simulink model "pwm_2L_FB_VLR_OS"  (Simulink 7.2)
settings: Solver=ode3  SolverMode=SingleTasking  StartTime=0.0  StopTime=0.1  FixedStep=10e-6  MaxStep=1e-4  RelTol=1e-3
PreLoadFcn:
  | INIT_PWM_2L

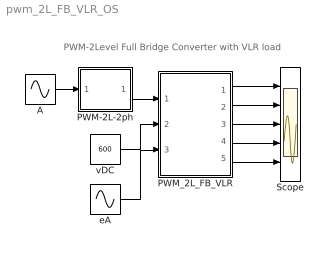
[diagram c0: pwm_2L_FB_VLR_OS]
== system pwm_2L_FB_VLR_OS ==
  note: PWM-2Level Full Bridge Converter with VLR load
  A : Sin  Amplitude=.8  Frequency=2*pi*50  Phase=[0 ]  SampleTime=0
  PWM-2L-2ph : Subsystem  mask(PWM-2L-2PH){FT=900, PHT=0, DT=1e-6}
      mask prompts: FT "Triangular Frequency"; PHT "Trian. Phase Angle (Degree)"; DT "Dead Time"
      mask help: Pulse Width Modulation for 2 Legs of 2-Level Converter
  PWM_2L_FB_VLR : Subsystem  mask(pwm_2L_FB_VLR_OS){RL=1, LL=1e-3}
      mask prompts: RL "Load R"; LL "Load L"
      mask help: Open Source 2-Level FB_PWM Converter with VLR load Input Vector u: u[0]= TD1.gate u[1]= TD2.gate u[2]= TD3.gate u[3]= TD4.gate u[4]= VDC u[5]= EL, Load Voltage Output Vector y: y[0]= Va.v, Output Voltage to middle point y[1]= Ia.I, Output AC Current y[2]= Vab.V, Output AC Voltage y[3]= T1.I y[4]= D1.I y[5]= T1.V y[6]= DC.I, Input DC Current Parameter Vector p: p[0]= RL p[1]= LL You can pause the simulation during running, change the Parameters you want and continue the Simulation
  Scope : Scope  NumInputPorts=5
  eA : Sin  Amplitude=100  Frequency=2*pi*50  Phase="[0  ]"  SampleTime=0
  vDC : Constant  Value=600  OutDataType=sfix(16)  OutScaling=2^0
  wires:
  A/1 -> PWM-2L-2ph/1(I1)
  PWM_2L_FB_VLR/1(vA) -> Scope/1
  vDC/1 -> PWM_2L_FB_VLR/2(vDC)
  PWM-2L-2ph/1(O1) -> PWM_2L_FB_VLR/1(Sw)
  eA/1 -> PWM_2L_FB_VLR/3(EA)
  PWM_2L_FB_VLR/2(iA1) -> Scope/2
  PWM_2L_FB_VLR/3(vAB) -> Scope/3
  PWM_2L_FB_VLR/4(iT1,iD1,vT1) -> Scope/4
  PWM_2L_FB_VLR/5(iDC) -> Scope/5

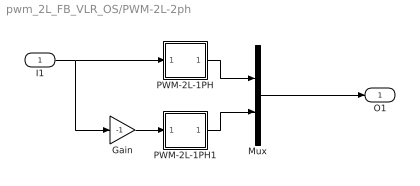
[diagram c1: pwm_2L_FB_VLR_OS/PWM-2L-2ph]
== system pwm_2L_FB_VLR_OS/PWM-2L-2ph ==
  I1 : Inport  OutDataType=sfix(16)  OutScaling=2^0
  Gain : Gain  Gain=-1  ParameterDataType=sfix(16)  ParameterScaling=2^0  OutDataType=sfix(16)  OutScaling=2^0
  Mux : Mux  Inputs=2
  PWM-2L-1PH : Subsystem  mask(PWM-2L-1PH){FT=FT, PHT=PHT, DT=DT}
      mask prompts: FT "Triangular Frequency"; PHT "Trian. Phase Angle (Degree)"; DT "Dead Time"
      mask help: Pulse Width Modulation for 1 Phase Converter
  PWM-2L-1PH1 : Subsystem  mask(PWM-2L-1PH){FT=FT, PHT=PHT, DT=DT}
      mask prompts: FT "Triangular Frequency"; PHT "Trian. Phase Angle (Degree)"; DT "Dead Time"
      mask help: Pulse Width Modulation for 1 Phase Converter
  O1 : Outport
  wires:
  Gain/1 -> PWM-2L-1PH1/1(In1)
  I1/1 -> Gain/1, PWM-2L-1PH/1(In1)
  PWM-2L-1PH/1(Out1) -> Mux/1
  PWM-2L-1PH1/1(Out1) -> Mux/2
  Mux/1 -> O1/1

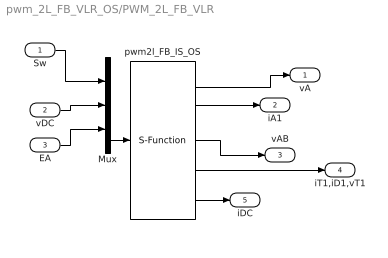
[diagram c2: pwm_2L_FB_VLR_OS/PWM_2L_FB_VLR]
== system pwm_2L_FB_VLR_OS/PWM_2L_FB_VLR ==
  Sw : Inport  OutDataType=sfix(16)  OutScaling=2^0
  vDC : Inport  Port=2  OutDataType=sfix(16)  OutScaling=2^0
  EA : Inport  Port=3  OutDataType=sfix(16)  OutScaling=2^0
  Mux : Mux  Inputs="[4  1  1]"
  pwm2l_FB_IS_OS : S-Function  FunctionName=s_pwm_2L_FB_VLR_OS  Parameters="[RL  LL]"  EnableBusSupport=off
  vA : Outport  OutDataType=sfix(16)  OutScaling=2^0
  iA1 : Outport  Port=2  OutDataType=sfix(16)  OutScaling=2^0
  vAB : Outport  Port=3  OutDataType=sfix(16)  OutScaling=2^0
  iT1,iD1,vT1 : Outport  Port=4  OutDataType=sfix(16)  OutScaling=2^0
  iDC : Outport  Port=5  OutDataType=sfix(16)  OutScaling=2^0
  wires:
  pwm2l_FB_IS_OS/4 -> iT1,iD1,vT1/1
  pwm2l_FB_IS_OS/3 -> vAB/1
  pwm2l_FB_IS_OS/2 -> iA1/1
  pwm2l_FB_IS_OS/1 -> vA/1
  EA/1 -> Mux/3
  Mux/1 -> pwm2l_FB_IS_OS/1
  vDC/1 -> Mux/2
  Sw/1 -> Mux/1
  pwm2l_FB_IS_OS/5 -> iDC/1

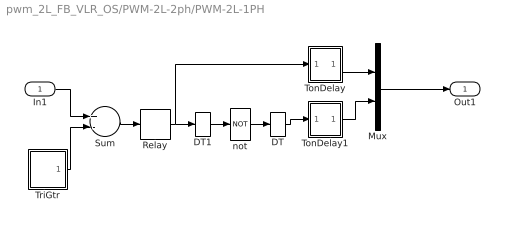
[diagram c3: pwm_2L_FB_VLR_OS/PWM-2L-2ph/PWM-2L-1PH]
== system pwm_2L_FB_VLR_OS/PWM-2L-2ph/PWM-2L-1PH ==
  In1 : Inport  OutDataType=sfix(16)  OutScaling=2^0
  DT : DataTypeConversion
  DT1 : DataTypeConversion
  Mux : Mux  Inputs=2
  Relay : Relay  OutDataType=sfix(16)  OutScaling=2^0
  Sum : Sum  Inputs=+-  OutDataType=sfix(16)  OutScaling=2^0
  TonDelay : Subsystem  mask(TonDelay){DT=DT}
      mask prompts: DT "Dead Time"
      mask help: Turn on dead time to protect against short circuit of the converter leg
  TonDelay1 : Subsystem  mask(TonDelay){DT=DT}
      mask prompts: DT "Dead Time"
      mask help: Turn on dead time to protect against short circuit of the converter leg
  TriGtr : Subsystem  mask(TriGtr){T=1/FT, Td=PHT/FT/360}
      mask prompts: T "Period Time"; Td "Time Delay"
      mask help: Triangular Wave Generator with variable time delay
  not : Logic  Operator=NOT  Inputs=1
  Out1 : Outport  InitialOutput=0
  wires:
  DT1/1 -> not/1
  DT/1 -> TonDelay1/1(s1)
  In1/1 -> Sum/1
  TriGtr/1(O) -> Sum/2
  Sum/1 -> Relay/1
  not/1 -> DT/1
  TonDelay1/1(s1d) -> Mux/2
  Relay/1 -> DT1/1, TonDelay/1(s1)
  TonDelay/1(s1d) -> Mux/1
  Mux/1 -> Out1/1

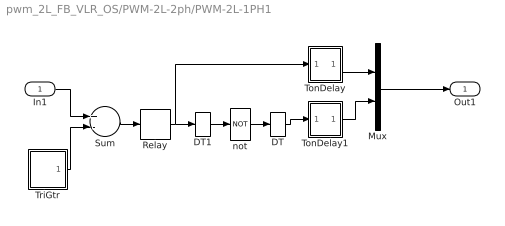
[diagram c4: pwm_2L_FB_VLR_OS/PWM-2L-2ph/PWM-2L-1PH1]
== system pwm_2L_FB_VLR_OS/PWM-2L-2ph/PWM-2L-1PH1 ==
  In1 : Inport  OutDataType=sfix(16)  OutScaling=2^0
  DT : DataTypeConversion
  DT1 : DataTypeConversion
  Mux : Mux  Inputs=2
  Relay : Relay  OutDataType=sfix(16)  OutScaling=2^0
  Sum : Sum  Inputs=+-  OutDataType=sfix(16)  OutScaling=2^0
  TonDelay : Subsystem  mask(TonDelay){DT=DT}
      mask prompts: DT "Dead Time"
      mask help: Turn on dead time to protect against short circuit of the converter leg
  TonDelay1 : Subsystem  mask(TonDelay){DT=DT}
      mask prompts: DT "Dead Time"
      mask help: Turn on dead time to protect against short circuit of the converter leg
  TriGtr : Subsystem  mask(TriGtr){T=1/FT, Td=PHT/FT/360}
      mask prompts: T "Period Time"; Td "Time Delay"
      mask help: Triangular Wave Generator with variable time delay
  not : Logic  Operator=NOT  Inputs=1
  Out1 : Outport  InitialOutput=0
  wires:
  Mux/1 -> Out1/1
  TonDelay/1(s1d) -> Mux/1
  Relay/1 -> TonDelay/1(s1), DT1/1
  TonDelay1/1(s1d) -> Mux/2
  not/1 -> DT/1
  Sum/1 -> Relay/1
  TriGtr/1(O) -> Sum/2
  In1/1 -> Sum/1
  DT/1 -> TonDelay1/1(s1)
  DT1/1 -> not/1

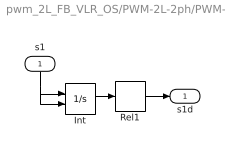
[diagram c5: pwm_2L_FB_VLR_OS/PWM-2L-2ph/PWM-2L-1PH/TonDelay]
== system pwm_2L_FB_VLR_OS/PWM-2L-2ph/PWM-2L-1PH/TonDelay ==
  s1 : Inport  Orientation=down  OutDataType=sfix(16)  OutScaling=2^0
  Int : Integrator  ExternalReset=falling
  Rel1 : Relay  OnSwitchValue=DT  OutDataType=sfix(16)  OutScaling=2^0
  s1d : Outport  InitialOutput=0
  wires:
  Int/1 -> Rel1/1
  s1/1 -> Int/2, Int/1
  Rel1/1 -> s1d/1

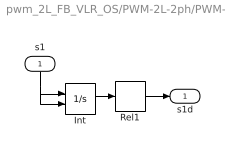
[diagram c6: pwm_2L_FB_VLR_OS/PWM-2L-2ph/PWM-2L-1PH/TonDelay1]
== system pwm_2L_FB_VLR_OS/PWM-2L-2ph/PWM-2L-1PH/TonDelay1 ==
  s1 : Inport  Orientation=down  OutDataType=sfix(16)  OutScaling=2^0
  Int : Integrator  ExternalReset=falling
  Rel1 : Relay  OnSwitchValue=DT  OutDataType=sfix(16)  OutScaling=2^0
  s1d : Outport  InitialOutput=0
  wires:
  Int/1 -> Rel1/1
  s1/1 -> Int/2, Int/1
  Rel1/1 -> s1d/1

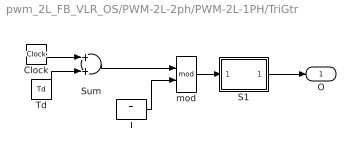
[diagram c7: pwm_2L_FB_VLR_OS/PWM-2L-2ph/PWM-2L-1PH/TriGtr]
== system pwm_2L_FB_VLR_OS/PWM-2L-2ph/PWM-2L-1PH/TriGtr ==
  Clock : Clock
  S1 : Subsystem
  Sum : Sum  OutDataType=sfix(16)  OutScaling=2^0
  T : Constant  Value=T  OutDataType=sfix(16)  OutScaling=2^0
  Td : Constant  Value=Td  OutDataType=sfix(16)  OutScaling=2^0
  mod : Math  Operator=mod
  O : Outport  InitialOutput=0
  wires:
  mod/1 -> S1/1(I1)
  S1/1(O1) -> O/1
  Clock/1 -> Sum/1
  T/1 -> mod/2
  Sum/1 -> mod/1
  Td/1 -> Sum/2

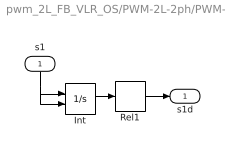
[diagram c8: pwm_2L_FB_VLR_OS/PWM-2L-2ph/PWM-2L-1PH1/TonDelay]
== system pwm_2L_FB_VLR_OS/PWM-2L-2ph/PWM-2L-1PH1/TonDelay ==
  s1 : Inport  Orientation=down  OutDataType=sfix(16)  OutScaling=2^0
  Int : Integrator  ExternalReset=falling
  Rel1 : Relay  OnSwitchValue=DT  OutDataType=sfix(16)  OutScaling=2^0
  s1d : Outport  InitialOutput=0
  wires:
  Rel1/1 -> s1d/1
  s1/1 -> Int/1, Int/2
  Int/1 -> Rel1/1

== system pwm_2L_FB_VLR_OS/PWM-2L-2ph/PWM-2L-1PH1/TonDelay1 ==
  s1 : Inport  Orientation=down  OutDataType=sfix(16)  OutScaling=2^0
  Int : Integrator  ExternalReset=falling
  Rel1 : Relay  OnSwitchValue=DT  OutDataType=sfix(16)  OutScaling=2^0
  s1d : Outport  InitialOutput=0
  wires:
  Rel1/1 -> s1d/1
  s1/1 -> Int/1, Int/2
  Int/1 -> Rel1/1

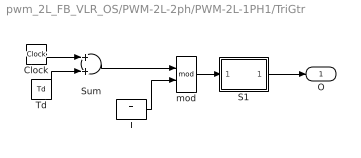
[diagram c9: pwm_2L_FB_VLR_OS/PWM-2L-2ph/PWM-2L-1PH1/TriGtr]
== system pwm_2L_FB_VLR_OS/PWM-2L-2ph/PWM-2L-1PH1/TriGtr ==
  Clock : Clock
  S1 : Subsystem
  Sum : Sum  OutDataType=sfix(16)  OutScaling=2^0
  T : Constant  Value=T  OutDataType=sfix(16)  OutScaling=2^0
  Td : Constant  Value=Td  OutDataType=sfix(16)  OutScaling=2^0
  mod : Math  Operator=mod
  O : Outport  InitialOutput=0
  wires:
  Td/1 -> Sum/2
  Sum/1 -> mod/1
  T/1 -> mod/2
  Clock/1 -> Sum/1
  S1/1(O1) -> O/1
  mod/1 -> S1/1(I1)

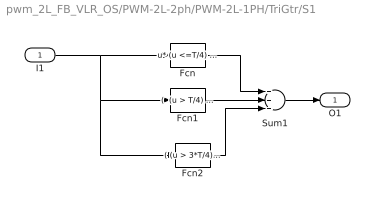
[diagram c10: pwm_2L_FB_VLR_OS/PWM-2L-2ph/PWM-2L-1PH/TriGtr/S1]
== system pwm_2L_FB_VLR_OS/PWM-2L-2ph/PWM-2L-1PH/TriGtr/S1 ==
  I1 : Inport  OutDataType=sfix(16)  OutScaling=2^0
  Fcn : Fcn  Expr=u* (u <=T/4) * 4/T
  Fcn1 : Fcn  Expr="(  (u > T/4) && ( u <=3*T/4) )* ( 1 - (u-T/4) *4/T )"
  Fcn2 : Fcn  Expr=( (u > 3*T/4)&& (u<=T)) * ( ((u -3*T/4)* 4/T )-1 )
  Sum1 : Sum  Inputs=+++  OutDataType=sfix(16)  OutScaling=2^0
  O1 : Outport
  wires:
  Fcn2/1 -> Sum1/3
  Fcn1/1 -> Sum1/2
  Fcn/1 -> Sum1/1
  Sum1/1 -> O1/1
  I1/1 -> Fcn/1, Fcn2/1, Fcn1/1

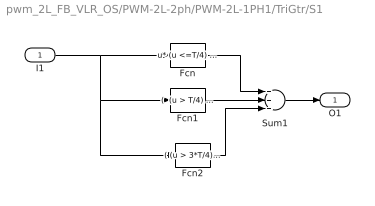
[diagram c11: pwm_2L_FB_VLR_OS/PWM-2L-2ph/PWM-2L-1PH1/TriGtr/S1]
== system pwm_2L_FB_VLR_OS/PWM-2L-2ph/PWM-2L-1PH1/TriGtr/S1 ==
  I1 : Inport  OutDataType=sfix(16)  OutScaling=2^0
  Fcn : Fcn  Expr=u* (u <=T/4) * 4/T
  Fcn1 : Fcn  Expr="(  (u > T/4) && ( u <=3*T/4) )* ( 1 - (u-T/4) *4/T )"
  Fcn2 : Fcn  Expr=( (u > 3*T/4)&& (u<=T)) * ( ((u -3*T/4)* 4/T )-1 )
  Sum1 : Sum  Inputs=+++  OutDataType=sfix(16)  OutScaling=2^0
  O1 : Outport
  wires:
  I1/1 -> Fcn1/1, Fcn2/1, Fcn/1
  Sum1/1 -> O1/1
  Fcn/1 -> Sum1/1
  Fcn1/1 -> Sum1/2
  Fcn2/1 -> Sum1/3
